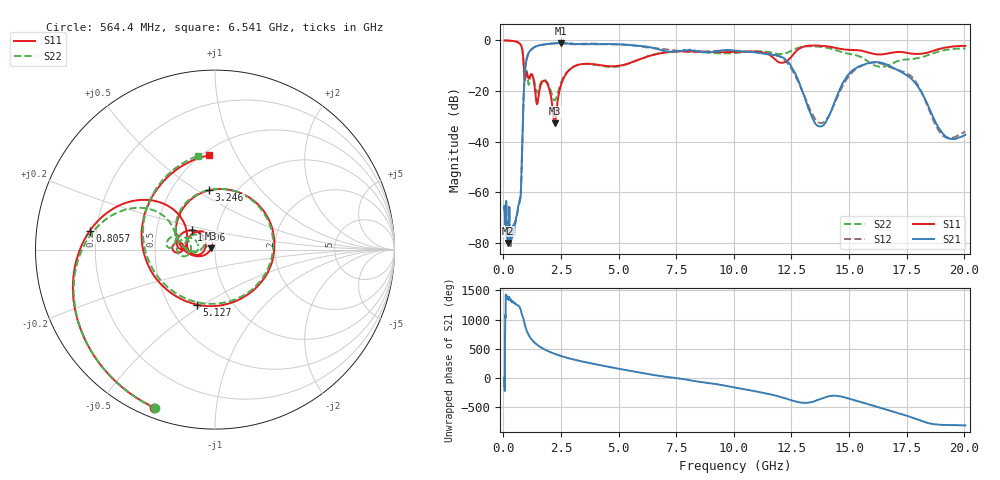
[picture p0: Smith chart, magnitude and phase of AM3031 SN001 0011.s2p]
# Hz S DB R 50
!freq MagS11 AngS11 MagS21 AngS21 MagS12 AngS12 MagS22 AngS22
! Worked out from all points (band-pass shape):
!   1601 points, 50 MHz to 20.05 GHz, reference 50 ohm
!   highest |S21| = -1.05 dB at 2.507 GHz (marker M1); lowest = -80.0 dB at 205.3 MHz (marker M2)
!   |S21| within 3 dB of the highest: 1.154 GHz to 6.925 GHz (5.77 GHz wide, 143 % of centre); 9.407 GHz to 10.09 GHz (686.8 MHz wide, 7.04 % of centre)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
!   lowest |S11| = -32.7 dB at 2.224 GHz (marker M3), VSWR 1.05, Z = 47.9 + j0.866 ohm
!   |S11| at or under -10 dB: 881.9 MHz to 3.117 GHz (2.235 GHz wide, 112 % of centre); 4.413 GHz to 4.994 GHz (581.5 MHz wide, 12.4 % of centre)
!   |S22| runs from -23.7 to 0.0 dB; largest |S21 - S12| = 0.068
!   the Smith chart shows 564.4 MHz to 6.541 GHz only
!   S11 on the Smith chart (normalised r, x): 564.4 MHz: 0.04, -0.68; 805.7 MHz: 0.17, +0.07; 1.306 GHz: 0.75, +0.17; 3.246 GHz: 0.76, +0.56; 5.127 GHz: 0.69, -0.47; 6.541 GHz: 0.54, +0.78
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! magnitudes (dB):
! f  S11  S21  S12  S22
! 50 MHz  0.0  -66.2  -68.1  0.0
! 135.9 MHz  0.0  -73.5  -75.0  0.0
! 205.3 MHz  -0.1  -80.0  -75.0  -0.1
! 250.4 MHz  -0.1  -66.4  -66.0  -0.1
! 369.6 MHz  -0.2  -77.5  -77.0  -0.2
! 564.4 MHz  -0.5  -69.3  -69.4  -0.5
! 733.7 MHz  -1.5  -62.3  -61.9  -1.5
! 805.7 MHz  -3.0  -44.8  -44.6  -3.2
! 1.005 GHz  -12.5  -7.4  -7.3  -12.0
! 1.306 GHz  -15.5  -2.8  -2.9  -14.9
! 1.886 GHz  -16.8  -1.5  -1.5  -16.3
! 2.224 GHz  -32.7  -1.1  -1.1  -23.6
! 2.507 GHz  -17.3  -1.1  -1.1  -16.5
! 2.722 GHz  -13.1  -1.1  -1.3  -12.9
! 3.246 GHz  -9.6  -1.4  -1.5  -9.6
! 5.127 GHz  -9.8  -1.6  -1.6  -10.0
! 6.541 GHz  -5.6  -3.1  -3.0  -5.5
! 7.402 GHz  -4.4  -4.3  -3.9  -4.4
! 11.91 GHz  -8.4  -6.1  -6.0  -5.3
! 13.73 GHz  -2.1  -33.9  -32.6  -2.5
! 16.44 GHz  -5.5  -8.9  -9.3  -10.4
! 20.05 GHz  -2.1  -37.3  -36.0  -3.1
